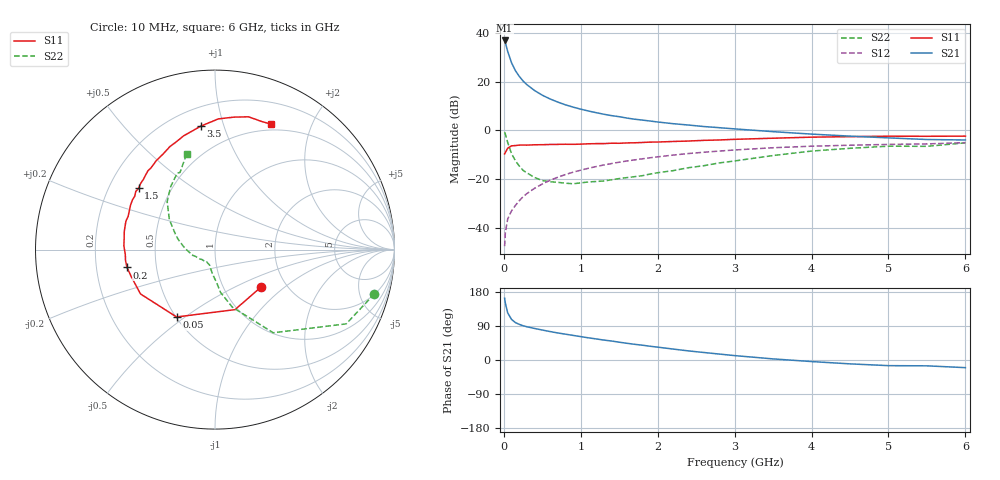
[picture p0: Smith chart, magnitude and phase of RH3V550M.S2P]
! SIEMENS Small Signal Semiconductors
! BFR106
! Si NPN RF Bipolar Junction Transistor in SOT23
! VCE = 3.5 V  IC = 50 mA
! Common Emitter S-Parameters:  August  1996
# GHz  S  MA  R  50
!  f  S11  S21  S12  S22
! GHz  MAG  ANG  MAG  ANG  MAG  ANG  MAG  ANG
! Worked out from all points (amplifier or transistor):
!   36 points, 10 MHz to 6 GHz, reference 50 ohm
!   highest |S21| = 37.0 dB at 10 MHz (marker M1)
!   |S21| within 3 dB of that: start of sweep to 37.29 MHz
!   unconditionally stable (mu >= 1): 246.3 MHz to 2.36 GHz
!   at 250 MHz: K = 1.00, MAG = 23.5 dB, |S12| = -27.3 dB
!   at 1.4 GHz: K = 1.05, MAG = 8.4 dB, |S12| = -13.6 dB
!   at 6 GHz: K = 0.99, MSG = 0.6 dB, |S12| = -5.0 dB
!   S11 on the Smith chart (normalised r, x): 10 MHz: 1.48, -0.70; 50 MHz: 0.50, -0.46; 200 MHz: 0.34, -0.09; 1.5 GHz: 0.33, +0.32; 3.5 GHz: 0.32, +0.84; 6 GHz: 0.43, +1.45
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0.01  0.3303 -39.6  70.62 163.1  0.0042 80.0  0.922 -15.5
0.02  0.3526 -71.6  63.34 149.7  0.008 70.2  0.84 -29.5
0.05  0.4321 -119.7  42.02 124.3  0.0152 60.4  0.5657 -55.0
0.1  0.4829 -149.2  24.61 107.1  0.0223 60.6  0.3353 -73.2
0.15  0.4903 -162.1  16.96 98.8  0.0288 64.3  0.2392 -82.8
0.2  0.5002 -168.5  12.97 94.1  0.036 67.7  0.1865 -86.9
0.25  0.5023 -173.1  10.4 90.4  0.0434 69.2  0.1516 -92.5
0.3  0.5004 -176.7  8.718 87.7  0.0506 70.5  0.1346 -96.2
0.4  0.5081 177.5  6.604 83.2  0.0649 71.3  0.108 -103.0
0.5  0.51 173.0  5.302 79.1  0.0795 71.5  0.0936 -107.8
0.6  0.5153 168.8  4.443 75.1  0.0947 71.1  0.0884 -112.4
0.7  0.5177 165.3  3.837 71.4  0.1092 70.2  0.086 -118.0
0.9  0.5182 159.0  3.018 64.9  0.1391 67.8  0.0804 -126.9
1.1  0.5323 152.1  2.51 58.5  0.1673 65.4  0.0877 -135.0
1.5  0.5456 141.2  1.918 47.0  0.223 59.6  0.1029 -150.4
1.7  0.5583 135.8  1.704 41.4  0.2486 56.6  0.1125 -159.4
2.2  0.5939 123.4  1.378 28.9  0.3118 48.8  0.1495 -176.4
2.8  0.6382 109.7  1.141 15.7  0.3775 39.3  0.2153 163.9
3.5  0.6931 96.4  0.945 2.9  0.4419 28.7  0.3056 146.4
4.5  0.7455 81.9  0.765 -10.2  0.4978 14.0  0.4301 125.0
5.5  0.7597 69.9  0.652 -15.4  0.5298 4.7  0.4719 114.4
6  0.7652 66.1  0.638 -20.2  0.5615 -2.3  0.5565 106.5
